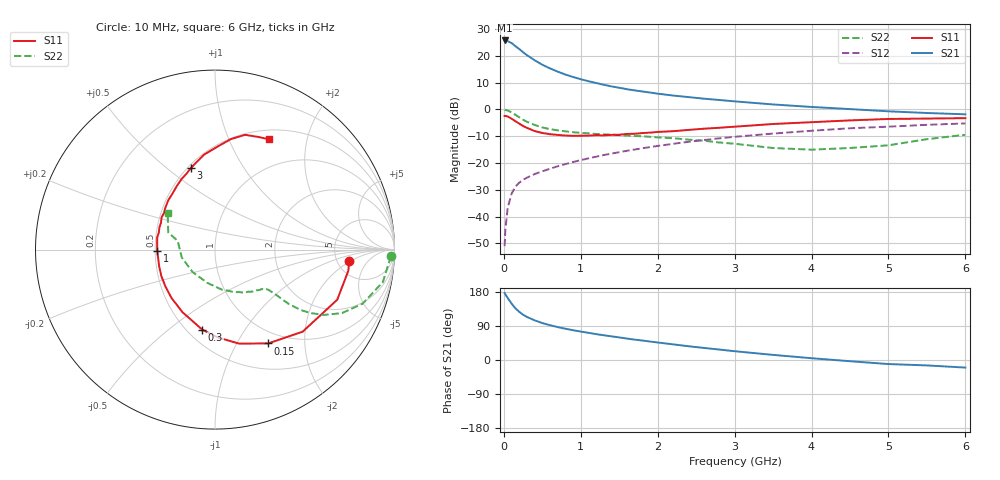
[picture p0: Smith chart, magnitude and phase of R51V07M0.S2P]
! SIEMENS Small Signal Semiconductors
! BFR183
! Si NPN RF Bipolar Junction Transistor in SOT23
! VCE = 1 V  IC = 7 mA
! Common Emitter S-Parameters:  May  1996
# GHz  S  MA  R  50
!  f  S11  S21  S12  S22
! GHz  MAG  ANG  MAG  ANG  MAG  ANG  MAG  ANG
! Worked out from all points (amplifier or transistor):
!   36 points, 10 MHz to 6 GHz, reference 50 ohm
!   highest |S21| = 25.7 dB at 10 MHz (marker M1)
!   |S21| within 3 dB of that: start of sweep to 190.9 MHz
!   unconditionally stable (mu >= 1): 835.2 MHz to 2.792 GHz
!   at 250 MHz: K = 0.53, MSG = 23.8 dB, |S12| = -26.3 dB
!   at 1.4 GHz: K = 1.07, MAG = 10.9 dB, |S12| = -16.5 dB
!   at 6 GHz: K = 0.93, MSG = 1.7 dB, |S12| = -5.3 dB
!   S11 on the Smith chart (normalised r, x): 10 MHz: 6.48, -1.82; 150 MHz: 0.83, -1.36; 300 MHz: 0.59, -0.66; 1 GHz: 0.51, -0.01; 3 GHz: 0.52, +0.61; 6 GHz: 0.61, +1.42
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0.01  0.7502 -4.7  19.26 176.9  0.0028 86.4  0.9817 -2.2
0.02  0.7522 -9.0  19.06 173.2  0.0058 85.0  0.9714 -4.4
0.05  0.736 -22.3  18.73 163.7  0.0144 80.5  0.9527 -10.9
0.1  0.6691 -43.1  17.22 149.0  0.0265 70.7  0.8763 -20.1
0.15  0.601 -60.4  15.08 136.5  0.036 64.4  0.7907 -26.6
0.2  0.5409 -75.6  13.33 127.1  0.0428 60.7  0.7087 -30.9
0.25  0.4894 -88.3  11.63 119.4  0.0484 57.6  0.6387 -33.6
0.3  0.4513 -99.1  10.24 113.6  0.0531 57.0  0.5868 -35.1
0.4  0.3932 -117.4  8.241 104.7  0.0619 56.3  0.5114 -36.4
0.5  0.3622 -132.2  6.789 97.4  0.0698 56.8  0.459 -36.5
0.6  0.3435 -143.9  5.794 91.8  0.0779 57.2  0.4265 -36.5
0.7  0.333 -154.0  5.05 86.8  0.0866 57.9  0.4055 -36.6
0.8  0.3247 -163.2  4.455 82.5  0.095 58.3  0.388 -36.8
1  0.3218 -179.0  3.644 75.0  0.1126 59.2  0.364 -37.4
1.1  0.3236 174.1  3.348 71.7  0.1218 59.4  0.3557 -38.6
1.6  0.3476 148.9  2.372 56.6  0.1683 57.8  0.3235 -44.5
2.2  0.3909 127.5  1.808 41.3  0.2272 53.4  0.2898 -55.8
3  0.4743 106.4  1.408 23.2  0.3072 44.8  0.2279 -79.7
3.5  0.5325 96.6  1.233 13.5  0.3528 38.5  0.1899 -103.4
4.5  0.6215 81.9  1.01 -3.2  0.4433 25.6  0.19 -166.5
5.5  0.6722 69.0  0.854 -14.3  0.5141 13.7  0.2775 159.8
6  0.6846 63.8  0.807 -20.0  0.5458 5.9  0.3349 142.0
